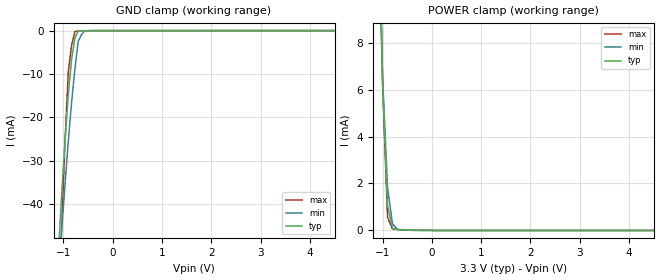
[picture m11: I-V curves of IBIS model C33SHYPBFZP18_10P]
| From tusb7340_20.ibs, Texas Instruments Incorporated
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|   Model Cell C33SHYPBFZP18_10P
|IC33SHYPBFZP18_PI_3P3
[Model]   C33SHYPBFZP18_10P
Model_type   Input
Polarity   Non-Inverting
Vinl =  0.8V
Vinh =  2V
C_comp   0.3896289p   0.315767p   0.4571448p
[Model Spec]
Vinl   0.8V   0.8V   0.8V
Vinh   2V   2V   2V
[Temperature Range]   25   125   -40
[Voltage Range]   3.3   2.97   3.63
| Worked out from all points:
|   GND clamp passes 1 mA (typ) near -0.74 V on its own axis
|   POWER clamp passes 1 mA (typ) near -0.89 V on its own axis
[POWER_clamp]
|   voltage   I(typ)   I(min)   I(max)
-3.3V     301.3mA    233.2mA    387.8mA
-1.033V   9.442mA    8.932mA    10.15mA
-1V       6.337mA    6.546mA    6.224mA
-900mV    1.056mA    1.857mA    562uA
-800mV    99.62uA    290.3uA    67.85uA
-700mV    32.23uA    46.94uA    44.59uA
-500mV    15.38uA    9.196uA    23.78uA
6.6V      0A         0A         0A
[GND_clamp]
|   voltage   I(typ)   I(min)   I(max)
-3.3V     -758.5mA   -699.4mA   -1.009A
-1.1V     -51.16mA   -56.66mA   -67.07mA
-1.033V   -37.54mA   -45.81mA   -44.83mA
-966.7mV  -25.31mA   -35.41mA   -25.6mA
-900mV    -14.48mA   -25.46mA   -9.398mA
-833.3mV  -6.552mA   -16.52mA   -3.322mA
-766.7mV  -1.754mA   -8.869mA   -210.3uA
-700mV    -81.77uA   -2.516mA   -62.56uA
-633.3mV  -47.18uA   -921.8uA   -49.46uA
-566.7mV  -25.83uA   -88.27uA   -37.19uA
6.6V      3.911uA    3.046uA    8.179uA
